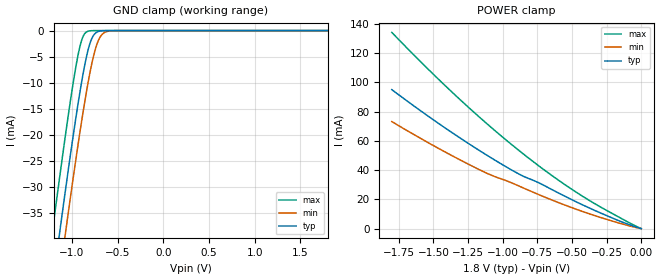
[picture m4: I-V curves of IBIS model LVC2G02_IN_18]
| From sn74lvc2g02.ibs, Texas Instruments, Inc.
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[Model]   LVC2G02_IN_18
Model_type  Input
Vinl=0.5775
Vinh=1.2675
| variable   typ   min   max
C_comp   5.00pF   NA   NA
[Temperature Range]   40   100   -40
| Ambient temperature   25   85   -40
[Voltage range]   1.8   1.65   1.95
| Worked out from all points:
|   GND clamp passes 1 mA (typ) near -0.77 V on its own axis
|   POWER clamp passes 1 mA (typ) near -0.03 V on its own axis
[GND Clamp]
| LVC2G02_IN_18
|   Voltage   I(typ)   I(min)   I(max)
-5.5V     -655.2mA   -662.2mA   -646.6mA
-1.215V   -49.6mA    -57.88mA   -38.96mA
-1.135V   -39.07mA   -47.36mA   -28.42mA
-1.075V   -31.35mA   -39.6mA    -20.75mA
-1.055V   -28.82mA   -37.05mA   -18.27mA
-955mV    -16.68mA   -24.66mA   -6.874mA
-885mV    -9.098mA   -16.55mA   -1.486mA
-825mV    -3.922mA   -10.26mA   -137.1uA
-780mV    -1.472mA   -6.227mA   -17.15uA
-715mV    -205.4uA   -2.128mA   -808.5nA
-650mV    -22.01uA   -443.9uA   -37.93nA
1.8V      3.326pA    6.142pA    3.026pA
[POWER Clamp]
| LVC2G02_IN_18
|   Voltage   I(typ)   I(min)   I(max)
-1.8V     95.04mA    73.2mA     134.2mA
-1.55V    77.73mA    59.44mA    110.2mA
-1.305V   61.82mA    46.88mA    88mA
-1.11V    49.98mA    37.68mA    71.43mA
-845mV    35.58mA    27.58mA    50.62mA
-750mV    31.82mA    23.7mA     43.68mA
-630mV    25.99mA    19.03mA    35.32mA
-430mV    16.56mA    11.94mA    22.54mA
-175mV    5.933mA    4.232mA    8.589mA
-16.28fV  7.417pA    238pA      400.9pA
